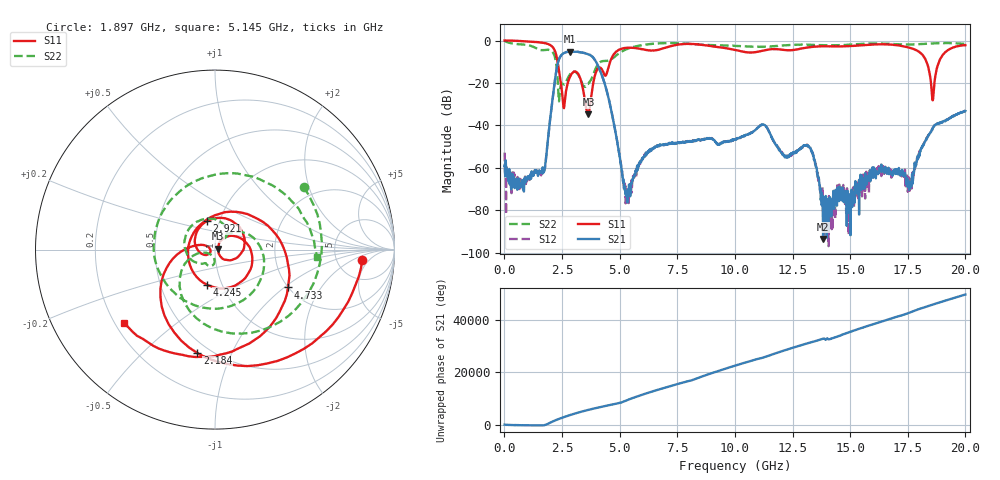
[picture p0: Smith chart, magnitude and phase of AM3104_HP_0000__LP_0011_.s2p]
!Created with skrf (http://scikit-rf.org).
# Hz S RI R 50.0
!freq ReS11 ImS11 ReS21 ImS21 ReS12 ImS12 ReS22 ImS22
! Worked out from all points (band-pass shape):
!   1601 points, 10 MHz to 20 GHz, reference 50 ohm
!   highest |S21| = -5.21 dB at 2.846 GHz (marker M1); lowest = -93.5 dB at 13.83 GHz (marker M2)
!   |S21| within 3 dB of the highest: 2.394 GHz to 3.861 GHz (1.468 GHz wide, 46.9 % of centre)
!   lowest |S11| = -34.8 dB at 3.646 GHz (marker M3), VSWR 1.04, Z = 51.8 + j0.505 ohm
!   |S11| at or under -10 dB: 2.309 GHz to 4.588 GHz (2.279 GHz wide, 66.1 % of centre); 18.31 GHz to 18.86 GHz (546.4 MHz wide, 2.94 % of centre)
!   |S22| runs from -28.7 to -0.2 dB; largest |S21 - S12| = 0.0044
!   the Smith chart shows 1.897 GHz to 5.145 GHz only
!   S11 on the Smith chart (normalised r, x): 1.897 GHz: 9.12, -3.20; 2.184 GHz: 0.43, -0.75; 2.921 GHz: 0.87, +0.28; 4.245 GHz: 0.85, -0.35; 4.733 GHz: 1.99, -1.06; 5.145 GHz: 0.24, -0.34
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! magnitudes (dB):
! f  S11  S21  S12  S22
! 10 MHz  0.0  -59.1  -52.9  -0.2
! 684.7 MHz  -0.2  -68.6  -67.0  -1.8
! 1.672 GHz  -1.1  -61.3  -62.4  -4.6
! 1.897 GHz  -1.7  -45.5  -45.7  -4.4
! 2.184 GHz  -4.7  -19.5  -19.5  -7.6
! 2.559 GHz  -30.9  -6.1  -6.1  -20.5
! 2.846 GHz  -17.1  -5.2  -5.2  -15.9
! 2.921 GHz  -15.7  -5.3  -5.3  -15.0
! 3.346 GHz  -19.8  -5.6  -5.6  -19.5
! 3.646 GHz  -34.8  -6.5  -6.6  -20.3
! 4.245 GHz  -13.9  -16.9  -16.9  -9.8
! 4.733 GHz  -6.8  -38.2  -38.2  -8.1
! 5.145 GHz  -3.7  -66.4  -64.3  -4.9
! 6.682 GHz  -4.3  -49.5  -49.6  -1.4
! 10.01 GHz  -4.4  -46.7  -46.5  -2.5
! 13.34 GHz  -3.0  -52.5  -52.4  -2.1
! 13.83 GHz  -2.7  -93.5  -83.1  -2.2
! 16.68 GHz  -1.8  -61.7  -62.0  -1.6
! 17.6 GHz  -3.5  -67.8  -69.2  -1.9
! 18.59 GHz  -28.2  -41.1  -41.3  -1.4
! 19.03 GHz  -6.7  -38.2  -38.0  -1.2
! 20 GHz  -2.2  -33.2  -33.2  -1.6
